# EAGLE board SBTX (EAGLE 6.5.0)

Size 45 x 59 mm. Coordinates in mm from the lower left corner, seen from the top.
Outline: 43,2 40,2 40,0 37,0 37,2 8,2 8,0 5,0 5,2 2,2 2,5 0,5 0,8 2,8 2,19.4 6.2,19.4 6.2,40.2 2,40.2 2,44 0,44 0,47 2,47 2,57.6 9,57.6 9,59 12,59 12,57.6 33,57.6 33,59 36,59 36,57.6 43,57.6 43,47 45,47 45,44 43,44 43,40.2 38.8,40.2 38.8,19.4 43,19.4 43,8 45,8 45,5 43,5 43,2
Copper layers (1*16): Top 0.018mm / dielectric 1.5mm / Bottom 0.018mm
Design rules "default": minimum track width 0.15mm, minimum drill 0.3mm, track to track 0.18mm, track to pad 0.18mm, pad to pad 0.18mm, via to via 0.18mm, smd to smd 0.18mm, copper to edge 40mil, drill to drill 8mil, minimum pad ring 0.15mm, minimum via ring 0.15mm, stop-mask expansion 4mil, vias tented up to drill 0.5mm, thermal gap 10mil
Net classes: 1 vcc: width 0.254 mm

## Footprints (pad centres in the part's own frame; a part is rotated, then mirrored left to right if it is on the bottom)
1X05 = drill 1.016 long: 1 -5.08,0; 2 -2.54,0; 3 0,0; 4 2.54,0; 5 5.08,0

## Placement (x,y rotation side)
JP7  [1X05]  6.19,9.58 90 bottom

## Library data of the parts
JP7 = pinhead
